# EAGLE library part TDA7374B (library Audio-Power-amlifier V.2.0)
The TDA7374B is a new technology class AB Audio Dual Bridge Power Amplifier in Multiwatt package designed for car radio applications. Thanks to the fully complementary PNP/NPN output configuration the high power performances of the TDA7374B are obtained without bootstrap capacitors.
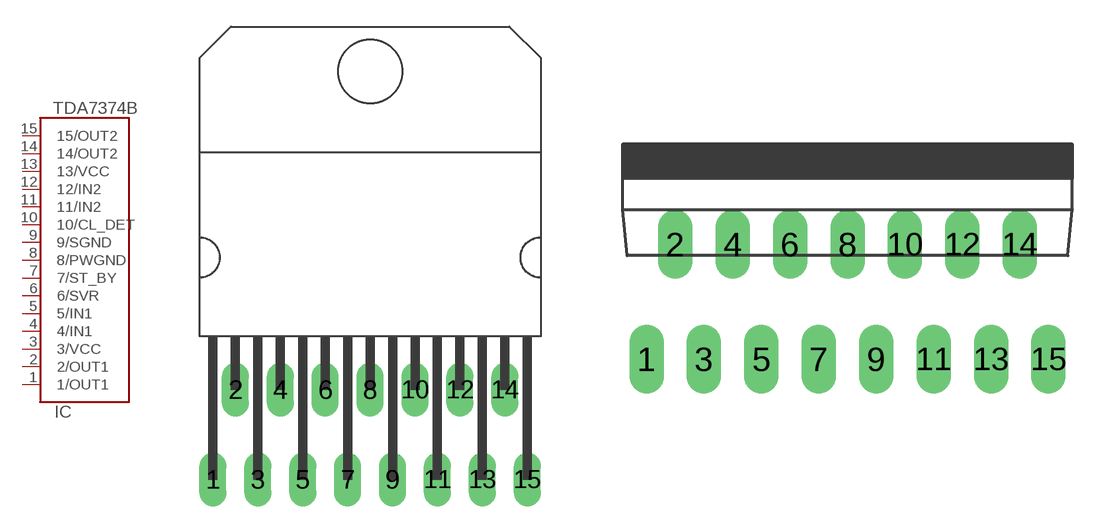
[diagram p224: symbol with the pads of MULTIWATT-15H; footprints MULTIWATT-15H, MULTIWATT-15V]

Designator prefix IC

## TDA7374BTDA7374BH  [MULTIWATT-15H]
1  1/OUT1  out
2  2/OUT1  out
3  3/VCC  pwr
4  4/IN1  in
5  5/IN1  in
6  6/SVR
7  7/ST_BY  in
8  8/PWGND  pwr
9  9/SGND  pwr
10  10/CL_DET
11  11/IN2  in
12  12/IN2  in
13  13/VCC  pwr
14  14/OUT2  out
15  15/OUT2  out

## TDA7374BTDA7374BV  [MULTIWATT-15V]
Pads as for MULTIWATT-15H

## Footprint MULTIWATT-15H (pad centres in mm)
Multiwatt 15 horizontal
drill 1.016 long: 1 -8.89,-5.08; 2 -7.62,0; 3 -6.35,-5.08; 4 -5.08,0; 5 -3.81,-5.08; 6 -2.54,0; 7 -1.27,-5.08; 8 0,0; 9 1.27,-5.08; 10 2.54,0; 11 3.81,-5.08; 12 5.08,0; 13 6.35,-5.08; 14 7.62,0; 15 8.89,-5.08

## Footprint MULTIWATT-15V (pad centres in mm)
Multiwatt 15 vertical
drill 1.016 long: 1 -8.89,-5.08; 2 -7.62,0; 3 -6.35,-5.08; 4 -5.08,0; 5 -3.81,-5.08; 6 -2.54,0; 7 -1.27,-5.08; 8 0,0; 9 1.27,-5.08; 10 2.54,0; 11 3.81,-5.08; 12 5.08,0; 13 6.35,-5.08; 14 7.62,0; 15 8.89,-5.08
